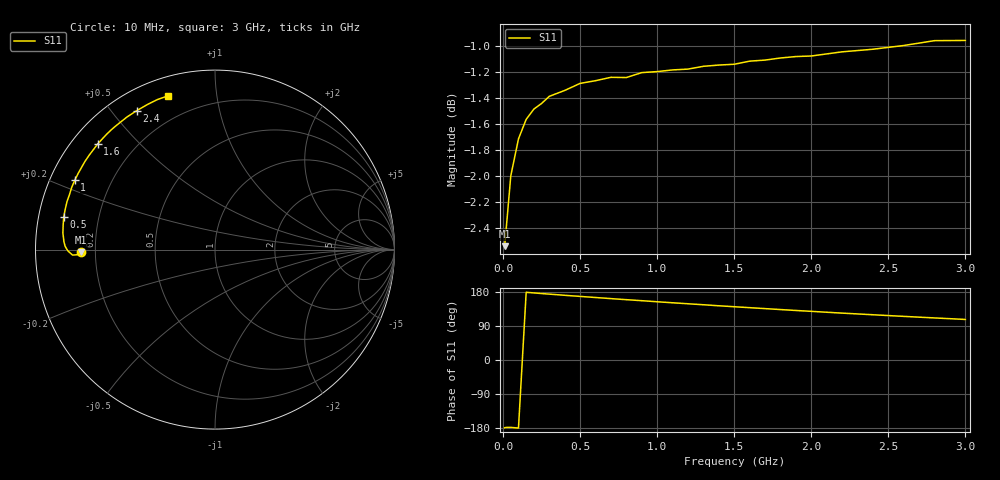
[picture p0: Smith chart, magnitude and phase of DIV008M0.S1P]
! SIEMENS Small Signal Semiconductors
! BAV99
! Silicon Switching Diode in SOT23
! IF = 8 mA
! S-Parameters:  May  1995
# GHz  S  MA  R  50
!  f  S11
! GHz  MAG  ANG
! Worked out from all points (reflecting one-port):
!   30 points, 10 MHz to 3 GHz, reference 50 ohm
!   lowest |S11| = -2.5 dB at 10 MHz (marker M1), VSWR 6.90, Z = 7.25 - j0.513 ohm
!   phase of S11 starts at -179 deg and turns -74 deg over the sweep
!   S11 on the Smith chart (normalised r, x): 10 MHz: 0.15, -0.01; 500 MHz: 0.07, +0.11; 1 GHz: 0.07, +0.23; 1.6 GHz: 0.07, +0.38; 2.4 GHz: 0.08, +0.58; 3 GHz: 0.09, +0.74
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0.01  0.7467 -178.8
0.02  0.7579 -177.9
0.05  0.7945 -177.8
0.1  0.821 -179.6
0.15  0.8353 178.7
0.2  0.8429 177.0
0.3  0.8525 173.8
0.4  0.8569 170.8
0.5  0.8623 167.8
0.6  0.8643 164.9
0.7  0.8669 162.0
0.8  0.8667 159.2
0.9  0.8705 156.5
1  0.8713 153.7
1.1  0.8726 151.0
1.2  0.8732 148.4
1.3  0.8754 145.8
1.4  0.8763 143.1
1.5  0.877 140.6
1.6  0.8794 138.1
1.8  0.8818 133.1
1.9  0.883 130.7
2  0.8834 128.4
2.2  0.8867 123.7
2.4  0.8887 119.4
2.6  0.8916 115.1
2.8  0.8955 111.0
3  0.8956 107.0
